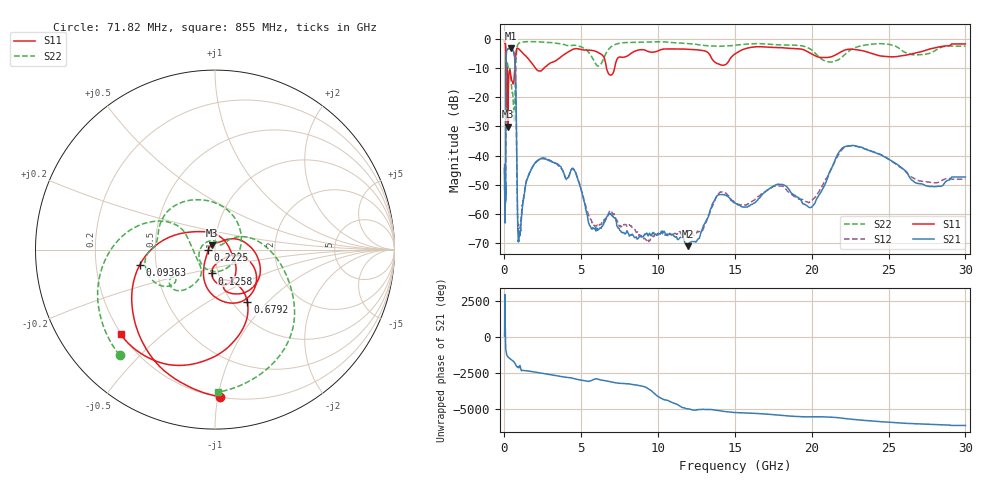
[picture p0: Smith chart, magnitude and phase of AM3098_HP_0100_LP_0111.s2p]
! Date/Time: Thu, Feb 28, 2019 8:35 AM
! Network Analyzer: Agilent Technologies E8364B Rev: A.07.50.67
! Sweep from 0.010 to 30.000 GHz, 1601 Points, Sweep Type: LOG
! Power Supply: 5.022 V, 0.002 A
# Hz S DB R 50
!freq MagS11 AngS11 MagS21 AngS21 MagS12 AngS12 MagS22 AngS22
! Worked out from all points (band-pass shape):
!   1601 points, 10 MHz to 30 GHz, reference 50 ohm
!   highest |S21| = -3.10 dB at 415.9 MHz (marker M1); lowest = -71.2 dB at 11.95 GHz (marker M2)
!   |S21| within 3 dB of the highest: 111.2 MHz to 660.4 MHz (549.2 MHz wide, 142 % of centre)
!   lowest |S11| = -30.0 dB at 229.3 MHz (marker M3), VSWR 1.06, Z = 48.2 + j2.48 ohm
!   |S11| at or under -10 dB: 176.5 MHz to 671.4 MHz (495 MHz wide, 117 % of centre); 2.041 GHz to 2.551 GHz (510.3 MHz wide, 22.2 % of centre); 6.648 GHz to 7.163 GHz (515.5 MHz wide, 7.46 % of centre)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
!   |S22| runs from -28.4 to -0.6 dB; largest |S21 - S12| = 0.012
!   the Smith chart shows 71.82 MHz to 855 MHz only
!   S11 on the Smith chart (normalised r, x): 71.82 MHz: 0.20, -1.02; 93.63 MHz: 0.40, -0.09; 125.8 MHz: 0.93, -0.25; 222.5 MHz: 0.93, -0.01; 679.2 MHz: 1.16, -0.77; 855 MHz: 0.20, -0.37
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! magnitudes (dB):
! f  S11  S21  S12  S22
! 10 MHz  -0.3  -46.4  -44.5  -0.6
! 38.04 MHz  -0.5  -60.1  -60.6  -0.9
! 71.82 MHz  -1.7  -53.8  -53.0  -2.0
! 93.63 MHz  -7.4  -21.9  -21.9  -8.6
! 125.8 MHz  -17.4  -4.6  -4.6  -10.3
! 144.7 MHz  -15.5  -3.8  -3.8  -10.7
! 184 MHz  -10.8  -3.6  -3.6  -8.0
! 222.5 MHz  -28.3  -3.2  -3.2  -9.3
! 229.3 MHz  -30.0  -3.2  -3.2  -9.5
! 415.9 MHz  -12.5  -3.1  -3.1  -13.1
! 550.5 MHz  -15.2  -3.8  -3.7  -19.3
! 679.2 MHz  -9.3  -7.2  -7.2  -21.6
! 747 MHz  -4.8  -17.9  -17.9  -8.0
! 855 MHz  -3.0  -63.1  -60.9  -2.0
! 2.084 GHz  -10.3  -42.1  -42.1  -0.8
! 4.503 GHz  -3.3  -44.7  -44.7  -2.0
! 7.926 GHz  -5.9  -66.6  -63.9  -1.1
! 11.95 GHz  -3.4  -71.2  -66.5  -1.4
! 14.09 GHz  -8.8  -53.5  -52.6  -2.3
! 20 GHz  -5.0  -57.8  -55.5  -3.6
! 22.56 GHz  -3.4  -36.6  -36.6  -3.5
! 30 GHz  -1.5  -47.4  -48.2  -2.3
